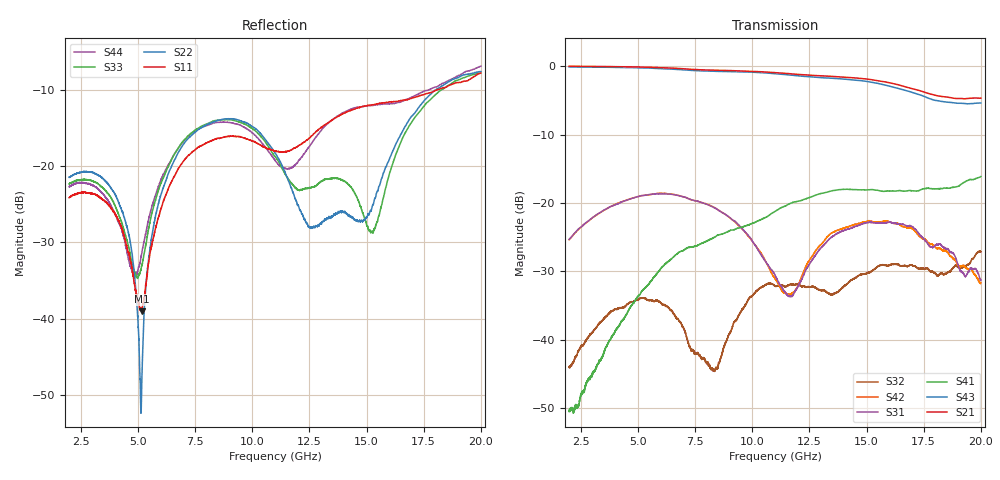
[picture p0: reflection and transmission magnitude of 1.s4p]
!Keysight Technologies,N5225A,MY51451420,A.10.40.12
!Date: Thursday, October 15, 2015 10:40:27
!Correction: S11(Full 4 Port(1,2,3,4))
!S12(Full 4 Port(1,2,3,4))
!S13(Full 4 Port(1,2,3,4))
!S14(Full 4 Port(1,2,3,4))
!S21(Full 4 Port(1,2,3,4))
!S22(Full 4 Port(1,2,3,4))
!S23(Full 4 Port(1,2,3,4))
!S24(Full 4 Port(1,2,3,4))
!S31(Full 4 Port(1,2,3,4))
!S32(Full 4 Port(1,2,3,4))
!S33(Full 4 Port(1,2,3,4))
!S34(Full 4 Port(1,2,3,4))
!S41(Full 4 Port(1,2,3,4))
!S42(Full 4 Port(1,2,3,4))
!S43(Full 4 Port(1,2,3,4))
!S44(Full 4 Port(1,2,3,4))
!S4P File: Measurements: <S11,S12,S13,S14>,
!<S21,S22,S23,S24>,
!<S31,S32,S33,S34>,
!<S41,S42,S43,S44>:
# Hz S  dB  R 50
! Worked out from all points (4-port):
!   6401 points, 2 GHz to 20 GHz, reference 50 ohm
!   strongest paths, dB at 2 GHz, 6.5 GHz, 11 GHz, 15.5 GHz, 20 GHz:
!     S21: 0.0, -0.3, -0.9, -2.1, -4.7
!     S43: -0.1, -0.4, -1.1, -2.5, -5.4
!     S41: -50.5, -28.1, -21.2, -18.1, -16.1
!     S31: -25.3, -18.7, -30.6, -22.9, -31.3
!     S42: -25.4, -18.7, -31.0, -22.8, -31.6
!     S32: -43.9, -35.8, -32.1, -29.2, -27.1
!   lowest |S11| = -39.1 dB at 5.173 GHz (marker M1), VSWR 1.02, Z = 49 - j0.522 ohm
!   |S11| at or under -10 dB: start of sweep to 18.11 GHz
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2e9  -24.16 43.2  0.02 -49.7  -25.32 39.1  -50.52 115.6
     0.02 -49.8  -21.48 41.6  -43.85 127.6  -25.34 39.6
     -25.30 39.1  -43.93 127.5  -22.37 40.9  -0.09 -50.2
     -50.46 117.2  -25.36 39.6  -0.09 -50.2  -22.73 30.9
4.30625e9  -28.21 -35.2  -0.06 -107.1  -19.83 -18.3  -37.19 -39.4
           -0.06 -107.1  -25.89 -21.2  -35.29 26.3  -19.80 -17.7
           -19.83 -18.3  -35.33 26.4  -27.52 -0.8  -0.17 -108.2
           -37.25 -39.4  -19.79 -17.7  -0.18 -108.2  -28.47 -52.0
5.1725e9  -39.06 -151.5  -0.12 -129.0  -18.93 -41.2  -32.89 -81.5
          -0.12 -129.1  -48.95 -172.4  -33.91 -8.8  -18.91 -40.3
          -18.92 -41.2  -33.92 -8.8  -33.06 76.8  -0.23 -130.3
          -32.89 -81.6  -18.91 -40.3  -0.23 -130.3  -31.53 179.5
6.688438e9  -20.85 105.1  -0.30 -167.5  -18.85 -82.6  -27.54 -151.3
            -0.29 -167.6  -18.75 98.1  -36.83 -70.4  -18.82 -81.6
            -18.84 -82.6  -36.83 -70.2  -18.04 87.5  -0.45 -169.2
            -27.51 -151.3  -18.82 -81.6  -0.46 -169.2  -18.05 100.0
1.044031e10  -17.42 17.8  -0.81 97.3  -27.82 -164.8  -22.33 83.3
             -0.81 97.2  -16.01 -4.4  -32.24 -83.9  -27.56 -163.3
             -27.82 -164.8  -32.26 -83.8  -16.35 2.8  -0.93 94.6
             -22.33 83.1  -27.56 -163.2  -0.94 94.6  -17.03 4.6
1.425688e10  -12.78 -29.2  -1.63 -2.6  -23.75 -148.4  -18.00 -38.6
             -1.63 -2.8  -26.60 -12.3  -31.48 -175.5  -23.38 -146.6
             -23.76 -148.4  -31.46 -175.1  -22.58 -1.4  -1.94 -6.5
             -18.00 -38.8  -23.38 -146.7  -1.94 -6.6  -12.63 -17.1
2e10  -7.81 74.0  -4.65 -151.0  -31.28 111.5  -16.10 165.8
      -4.65 -151.2  -7.62 89.5  -27.11 35.8  -31.66 130.7
      -31.28 111.5  -27.12 36.4  -7.82 76.5  -5.35 -153.3
      -16.12 165.7  -31.64 130.3  -5.36 -153.3  -6.93 73.1
